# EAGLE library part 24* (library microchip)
Serial EEPROM I2C
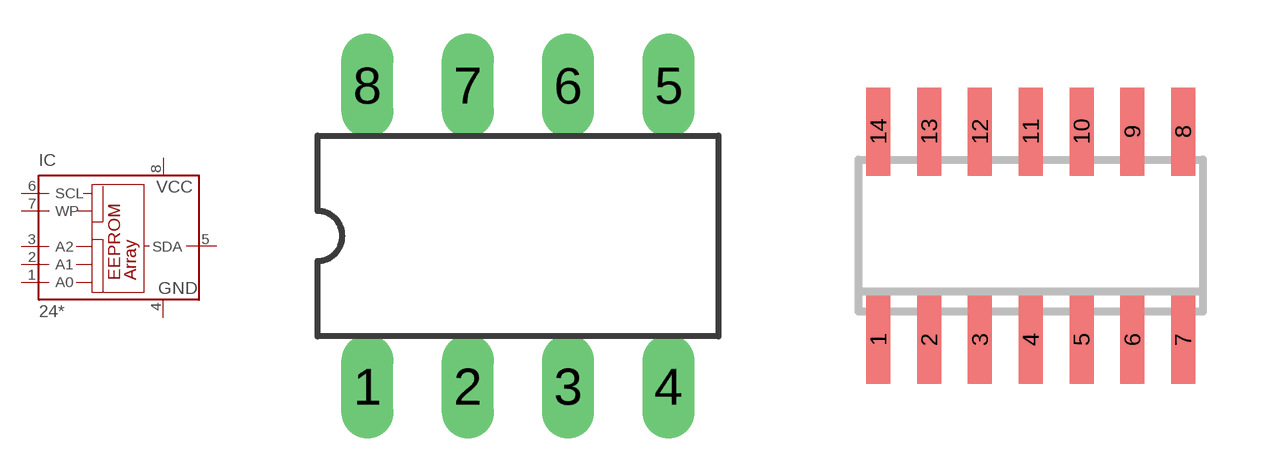
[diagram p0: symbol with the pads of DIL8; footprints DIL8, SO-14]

Designator prefix IC

## 24P, 24AA01P (MPN: 24AA01-I/P; OC_FARNELL: 1331266; OC_NEWARK: 35M0692), 24AA02P (MPN: 24AA02-I/P; OC_FARNELL: 1331271; OC_NEWARK: 95M2072), 24AA04P (MPN: 24AA04-I/P; OC_FARNELL: 1331275; OC_NEWARK: 35M0696), 24AA08P (MF: MICROCHIP; MPN: 24AA08-I/P; OC_FARNELL: 1331281; OC_NEWARK: 92C6825), 24AA128P (MF: MICROCHIP; MPN: 24AA128-I/P; OC_FARNELL: unknown; OC_NEWARK: 92C6840), 24AA16P (MPN: 24AA16-I/P; OC_FARNELL: 1331287; OC_NEWARK: 35M0705), 24AA256P (MF: MICROCHIP; MPN: 24AA256-I/P; OC_FARNELL: 1331294; OC_NEWARK: 92C6872), 24AA32AP (MF: MICROCHIP; MPN: 24AA32A-I/P; OC_FARNELL: 1331297; OC_NEWARK: 92C6885), 24AA64P (MF: MICROCHIP; MPN: 24AA64-I/P; OC_FARNELL: 1331303; OC_NEWARK: 92C6909), 24C01AP (MPN: M24C01-WBN6P; OC_FARNELL: 9882782; OC_NEWARK: 24M5067), 24C02AP (MF: MICROCHIP; MPN: 24C02C-I/P; OC_FARNELL: 1755843; OC_NEWARK: 96K4062), 24C04AP (MF: RAMTRON INTERNATIONAL CORP; MPN: FM24C04A-P; OC_FARNELL: 1094258; OC_NEWARK: 97H6447), 24C08BP (MPN: AT24C08B-PU; OC_FARNELL: 1362644; OC_NEWARK: 50M3317), 24C16BP (MPN: AT24C16B-PU; OC_FARNELL: 1362650; OC_NEWARK: 50M3323), 24C32AP (MPN: AT24C32C-PU; OC_FARNELL: 1362652; OC_NEWARK: 50M3325), 24C64P (MF: RAMTRON INTERNATIONAL CORP; MPN: FM24C64-P; OC_FARNELL: 1362657; OC_NEWARK: 97H6452), 24CL04BP (OC_FARNELL: unknown; OC_NEWARK: unknown), 24LC01P (MPN: 24LC01BH-I/P; OC_FARNELL: 1200025; OC_NEWARK: 77M3542), 24LC024P (MPN: 24LC024-I/P; OC_FARNELL: 1331317; OC_NEWARK: 35M0731), 24LC025P (MF: MICROCHIP; MPN: 24LC025-I/P; OC_FARNELL: unknown; OC_NEWARK: 92C7098), 24LC04P (MF: MICROCHIP; MPN: 24LC04B-I/P; OC_FARNELL: 1196811; OC_NEWARK: 62K0576), 24LC08BP (MF: MICROCHIP; MPN: 24LC08B/P; OC_FARNELL: 1084245; OC_NEWARK: 96K4073), 24LC128P (MF: MICROCHIP; MPN: 24LC128-I/P; OC_FARNELL: 9757929; OC_NEWARK: 12C2007), 24LC16BP (MF: MICROCHIP; MPN: 24LC16B/P; OC_FARNELL: 1200026; OC_NEWARK: 69K7671), 24LC256P (MF: MICROCHIP; MPN: 24LC256-E/P; OC_FARNELL: 9757970; OC_NEWARK: 92C7169), 24LC32AP (MF: MICROCHIP; MPN: 24LC32A/P; OC_FARNELL: 1084246; OC_NEWARK: 75K1884), 24LC64P (MF: MICROCHIP; MPN: 24LC64-I/P; OC_FARNELL: 9758054; OC_NEWARK: 62K0584), 24LCS52P (MF: MICROCHIP; MPN: 24LCS52-I/PG; OC_FARNELL: unknown; OC_NEWARK: 89H3098)  [DIL8]
1  A0  in
2  A1  in
3  A2  in
4  GND  pwr
5  SDA
6  SCL  in
7  WP  in
8  VCC  pwr

## 24SL, 24AA04SL (OC_FARNELL: unknown; OC_NEWARK: unknown), 24AA08SL (OC_FARNELL: unknown; OC_NEWARK: unknown), 24AA16SL (OC_FARNELL: unknown; OC_NEWARK: unknown), 24C01ASL (OC_FARNELL: unknown; OC_NEWARK: unknown), 24C02ASL (OC_FARNELL: unknown; OC_NEWARK: unknown), 24C04ASL (OC_FARNELL: unknown; OC_NEWARK: unknown), 24C08BSL (OC_FARNELL: unknown; OC_NEWARK: unknown), 24C16BSL (OC_FARNELL: unknown; OC_NEWARK: unknown), 24CL04ASL (OC_FARNELL: unknown; OC_NEWARK: unknown), 24LC08BSL (OC_FARNELL: unknown; OC_NEWARK: unknown), 24LC16BSL (OC_FARNELL: unknown; OC_NEWARK: unknown)  [SO-14]
2  A0  in
3  A1  in
5  A2  in
6  GND  pwr
9  SDA
10  SCL  in
12  WP  in
13  VCC  pwr

## 24SM, 24AA01SM (MF: MICROCHIP; MPN: 24AA01-I/SN; OC_FARNELL: 1331268; OC_NEWARK: 92C6793), 24AA02SM (MF: MICROCHIP; MPN: 24AA02-I/SN; OC_FARNELL: 1331272; OC_NEWARK: 92C6803), 24AA04SM (MF: MICROCHIP; MPN: 24AA04-I/SN; OC_FARNELL: 1331276; OC_NEWARK: 92C6814), 24AA08SM (MF: MICROCHIP; MPN: 24AA08-I/SN; OC_FARNELL: 1331282; OC_NEWARK: 92C6826), 24AA128SM (MF: MICROCHIP; MPN: 24AA128-I/MS; OC_FARNELL: 1331285; OC_NEWARK: 92C6839), 24AA16SM (MF: MICROCHIP; MPN: 24AA16-I/SN; OC_FARNELL: 1331289; OC_NEWARK: 96K4056), 24AA32ASM (MF: MICROCHIP; MPN: 24AA32A-I/SN; OC_FARNELL: 1617659; OC_NEWARK: 83C5815), 24C01ASM (MF: MICROCHIP; MPN: 24C01C/SN; OC_FARNELL: 1362638; OC_NEWARK: 96K4061), 24C02ASM (MF: MICROCHIP; MPN: 24C02C/SN; OC_FARNELL: 1084339; OC_NEWARK: 96K4065), 24C04ASM (MPN: M24C04-WMN6P; OC_FARNELL: 9882812; OC_NEWARK: 83K1376), 24C08BSM (MPN: AT24C08BN-SH-B; OC_FARNELL: 1362645; OC_NEWARK: 50M3318), 24C32ASM (MPN: IS24C32A-2GLI; OC_FARNELL: 1718129; OC_NEWARK: 43M4588), 24C64SM (MF: RAMTRON INTERNATIONAL CORP; MPN: FM24C64-S; OC_FARNELL: 9882685; OC_NEWARK: 98H0189), 24CL04BSM (MPN: FM24CL04-S; OC_FARNELL: 1607928; OC_NEWARK: 97H6443), 24LC08BSM (MF: MICROCHIP; MPN: 24LC08BT-I/SN; OC_FARNELL: 1818714; OC_NEWARK: 92C7127), 24LC128SM (MF: MICROCHIP; MPN: 24LC128-I/SM; OC_FARNELL: 9757937; OC_NEWARK: 92C7134), 24LC16BSM (MF: MICROCHIP; MPN: 24LC16B/SN; OC_FARNELL: 9757945; OC_NEWARK: 12C2012), 24LC32ASM (MF: MICROCHIP; MPN: 24LC32A/SM; OC_FARNELL: 1212670; OC_NEWARK: 96K4080), 24LC64SM (MF: MICROCHIP; MPN: 24LC64T-I/SN; OC_FARNELL: 9758070; OC_NEWARK: 12C2021)  [SO-08M]
Pads as for DIL8

## 24SN, 24AA01SN (MF: MICROCHIP; MPN: 24AA01/SN; OC_FARNELL: 1331268; OC_NEWARK: 89C9792), 24AA02SN (MPN: 24AA02/SN; OC_FARNELL: 1331272; OC_NEWARK: 89C9793), 24AA04SN (MF: MICROCHIP; MPN: 24AA04/SN; OC_FARNELL: 1331276; OC_NEWARK: 92C6818), 24AA08SN (MF: MICROCHIP; MPN: 24AA08-I/SN; OC_FARNELL: 1579568; OC_NEWARK: 92C6826), 24AA128SN (MF: MICROCHIP; MPN: 24AA128-I/SN; OC_FARNELL: unknown; OC_NEWARK: 92C6842), 24AA16SN (MF: MICROCHIP; MPN: 24AA16-I/SN; OC_FARNELL: 1331289; OC_NEWARK: 96K4056), 24AA256SN (MPN: 24AA256T-I/SM; OC_FARNELL: 1579570; OC_NEWARK: 08N6838), 24AA32ASN (MF: MICROCHIP; MPN: 24AA32A-I/SN; OC_FARNELL: 1617659; OC_NEWARK: 83C5815), 24AA64SN (MF: MICROCHIP; MPN: 24AA64-I/SN; OC_FARNELL: 1331304; OC_NEWARK: 85C2288), 24C08BSN (MPN: AT24C08BN-SH-B; OC_FARNELL: 1362645; OC_NEWARK: 50M3318), 24C16BSN (MPN: AT24C16BN-SH-B; OC_FARNELL: 1362651; OC_NEWARK: 50M3324), 24C32ASN (MPN: IS24C32A-2GLI; OC_FARNELL: 1224413; OC_NEWARK: 43M4588), 24CL04BSN (MF: RAMTRON INTERNATIONAL CORP; MPN: FM24CL04-G; OC_FARNELL: 1607928; OC_NEWARK: 10J0444), 24LC024SN (MF: MICROCHIP; MPN: 24LC024/SN; OC_FARNELL: 1659744; OC_NEWARK: 92C7092), 24LC025SN (MF: MICROCHIP; MPN: 24LC025/SN; OC_FARNELL: unknown; OC_NEWARK: 92C7103), 24LC08BSN (MPN: 24LC08B/SN; OC_FARNELL: 1212669; OC_NEWARK: 12C2005), 24LC128SN (MF: MICROCHIP; MPN: 24LC128-I/SNG; OC_FARNELL: 9757937; OC_NEWARK: 30H1511), 24LC16BSN (MF: MICROCHIP; MPN: 24LC16B/SN; OC_FARNELL: 9757945; OC_NEWARK: 12C2012), 24LC256SN (MF: MICROCHIP; MPN: 24LC256-I/SN; OC_FARNELL: 9757996; OC_NEWARK: 27C9144), 24LC32ASN (MF: MICROCHIP; MPN: 24LC32A/SN; OC_FARNELL: 9758003; OC_NEWARK: 33C2976), 24LC64SN (MF: MICROCHIP; MPN: 24LC64-I/SN; OC_FARNELL: 9758070; OC_NEWARK: 12C2020), 24LCS52SN (MF: MICROCHIP; MPN: 24LCS52-I/SN; OC_FARNELL: 1816066; OC_NEWARK: 92C7032)  [SO-08]
Pads as for DIL8

## 24ST, 24AA128ST (MF: MICROCHIP; MPN: 24AA128-I/ST; OC_FARNELL: unknown; OC_NEWARK: 92C6843), 24AA64ST (MPN: 25AA640A-I/ST; OC_FARNELL: 1818513; OC_NEWARK: 27M1300), 24C64ST (MPN: CAT24C64YI-GT3; OC_FARNELL: 1718133; OC_NEWARK: 08R5418), 24LC024ST (MPN: 24LC024H-I/ST; OC_FARNELL: 1659745; OC_NEWARK: 77M3584), 24LC025ST (MF: MICROCHIP; MPN: 24LC025-I/ST; OC_FARNELL: unknown; OC_NEWARK: 92C7100), 24LC128ST (MF: MICROCHIP; MPN: 24LC128-I/ST; OC_FARNELL: 1296573; OC_NEWARK: 62K0578), 24LC64ST (MF: MICROCHIP; MPN: 24LC64X-I/ST; OC_FARNELL: 1296582; OC_NEWARK: 96K4081), 24LCS52ST (MF: MICROCHIP; MPN: 24LCS52T/ST; OC_FARNELL: unknown; OC_NEWARK: 92C7040)  [TSSOP8]
Pads as for DIL8

## Footprint DIL8 (pad centres in mm)
Dual In Line package type P
drill 0.813 long: 1 -3.81,-3.81; 2 -1.27,-3.81; 3 1.27,-3.81; 4 3.81,-3.81; 5 3.81,3.81; 6 1.27,3.81; 7 -1.27,3.81; 8 -3.81,3.81

## Footprint SO-14 (pad centres in mm)
Small Outline Narrow Plastic Gull Wing 150-mil body, package type SL
smd 0.6 x 2.2: 1 -3.81,-2.6; 2 -2.54,-2.6; 3 -1.27,-2.6; 4 0,-2.6; 5 1.27,-2.6; 6 2.54,-2.6; 7 3.81,-2.6; 8 3.81,2.6; 9 2.54,2.6; 10 1.27,2.6; 11 0,2.6; 12 -1.27,2.6; 13 -2.54,2.6; 14 -3.81,2.6

## Footprint SO-08M (pad centres in mm)
Small Outline Medium Plastic Gull Wing 207-mil body, package type SM
smd 0.6 x 2.2: 1 -1.905,-3.33; 2 -0.635,-3.33; 3 0.635,-3.33; 4 1.905,-3.33; 5 1.905,3.33; 6 0.635,3.33; 7 -0.635,3.33; 8 -1.905,3.33

## Footprint SO-08 (pad centres in mm)
Small Outline Narrow Plastic Gull Wing 150-mil body, package type SN
smd 0.6 x 2.2: 1 -1.905,-2.6; 2 -0.635,-2.6; 3 0.635,-2.6; 4 1.905,-2.6; 5 1.905,2.6; 6 0.635,2.6; 7 -0.635,2.6; 8 -1.905,2.6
